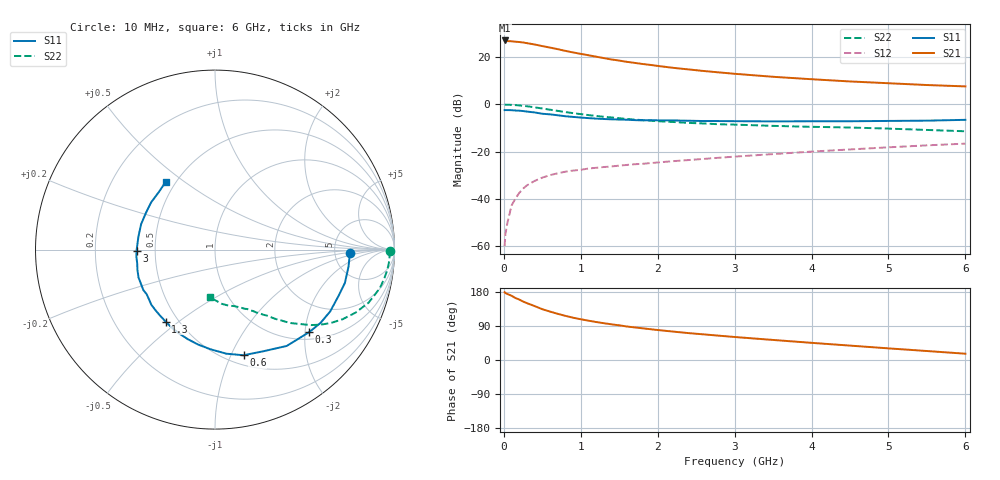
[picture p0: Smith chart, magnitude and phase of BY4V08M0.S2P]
! SIEMENS Small Signal Semiconductors
! BFY420
! Si NPN RF SIEGET Grounded Emitter Transistor in MICRO-X
! VCE = 4 V  IC = 8 mA
! Common Emitter S-Parameters:  October  1996
# GHz  S  MA  R  50
!  f  S11  S21  S12  S22
! GHz  MAG  ANG  MAG  ANG  MAG  ANG  MAG  ANG
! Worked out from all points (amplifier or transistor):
!   36 points, 10 MHz to 6 GHz, reference 50 ohm
!   highest |S21| = 26.9 dB at 10 MHz (marker M1)
!   |S21| within 3 dB of that: start of sweep to 598.9 MHz
!   unconditionally stable (mu >= 1): start of sweep to 13.81 MHz; 2.708 GHz to end of sweep
!   at 250 MHz: K = 0.22, MSG = 30.9 dB, |S12| = -35.7 dB
!   at 1.4 GHz: K = 0.68, MSG = 22.6 dB, |S12| = -26.3 dB
!   at 6 GHz: K = 1.09, MAG = 10.2 dB, |S12| = -16.7 dB
!   S11 on the Smith chart (normalised r, x): 10 MHz: 6.93, -0.66; 300 MHz: 1.17, -2.10; 600 MHz: 0.60, -1.12; 1.3 GHz: 0.43, -0.45; 3 GHz: 0.39, -0.01; 6 GHz: 0.44, +0.43
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0.01  0.7499 -1.6  22.19 179.0  0.001 22.3  0.9744 -0.5
0.02  0.7508 -3.0  22.08 176.8  0.0018 43.0  0.973 -1.2
0.05  0.75 -7.2  21.48 173.8  0.0033 68.4  0.9742 -3.3
0.1  0.7471 -14.4  21.33 169.6  0.0072 78.0  0.9665 -6.8
0.15  0.7348 -20.7  20.85 163.6  0.0101 73.0  0.9554 -10.1
0.2  0.7284 -28.2  20.57 159.6  0.0133 73.0  0.9429 -13.2
0.25  0.716 -34.8  20.11 154.4  0.0164 69.3  0.9226 -16.2
0.3  0.6977 -41.2  19.46 150.0  0.0193 69.5  0.9052 -19.1
0.4  0.6693 -53.3  18.27 142.3  0.0239 64.2  0.8578 -24.2
0.5  0.6274 -64.5  16.87 134.0  0.0281 59.9  0.8102 -28.6
0.6  0.6096 -74.9  15.7 127.8  0.0317 57.7  0.7648 -32.3
0.8  0.556 -92.5  13.37 116.5  0.0375 51.8  0.6814 -38.1
0.9  0.538 -99.8  12.39 111.6  0.0395 50.5  0.6467 -40.1
1.1  0.5076 -113.6  10.81 103.8  0.0437 48.7  0.5881 -44.1
1.3  0.4861 -124.5  9.408 97.1  0.047 47.7  0.5419 -46.8
1.7  0.4605 -143.0  7.458 86.0  0.0538 47.0  0.472 -51.5
2.2  0.4537 -159.9  5.864 75.0  0.0625 46.1  0.4207 -56.5
3  0.4373 -179.1  4.386 60.7  0.0779 44.6  0.3701 -63.1
3.5  0.4327 170.4  3.789 52.9  0.0882 43.1  0.348 -67.2
4.5  0.4358 152.1  3.021 38.0  0.1105 38.3  0.3215 -76.3
5.5  0.4486 133.9  2.538 23.7  0.1349 31.6  0.2854 -88.6
6  0.4669 126.1  2.375 16.6  0.1468 27.9  0.2676 -96.2
